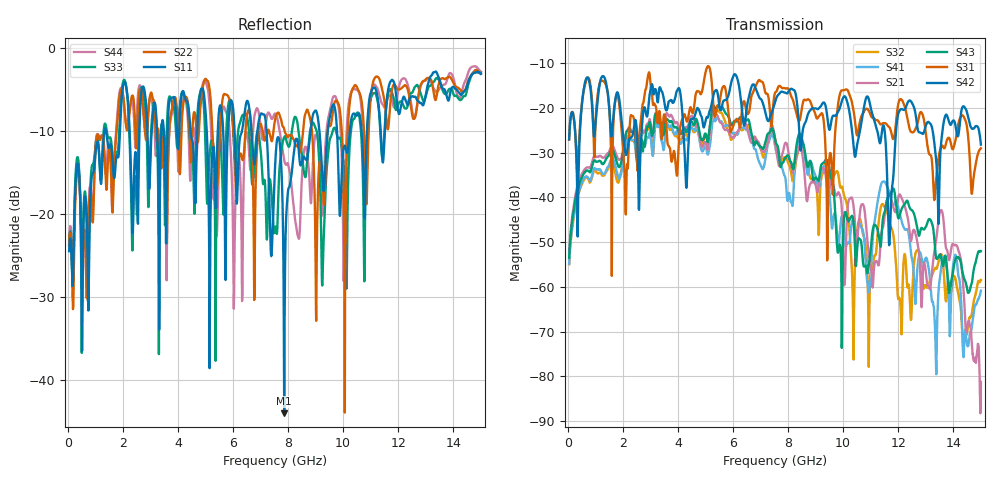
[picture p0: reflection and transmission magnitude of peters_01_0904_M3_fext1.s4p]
# MHZ S RI R 50.00
! FREQ  S11  S12  S13  S14
!  S21  S22  S23  S24
!  S31  S32  S33  S34
!  S41  S42  S43  S44
!  REAL  IMAG  REAL  IMAG  REAL  IMAG  REAL  IMAG
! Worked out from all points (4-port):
!   1496 points, 50 MHz to 15 GHz, reference 50 ohm
!   strongest paths, dB at 50 MHz, 3.79 GHz, 7.53 GHz, 11.27 GHz, 15 GHz:
!     S42: -27.0, -18.6, -18.6, -26.0, -28.2
!     S31: -27.1, -31.7, -16.5, -22.8, -29.0
!     S43: -53.5, -23.1, -27.1, -47.7, -52.0
!     S21: -52.9, -21.9, -28.1, -55.1, -81.3
!     S41: -54.9, -24.4, -28.5, -40.3, -60.9
!     S32: -55.0, -24.9, -26.9, -46.7, -58.5
!   lowest |S11| = -44.0 dB at 7.86 GHz (marker M1), VSWR 1.01, Z = 49.6 + j0.459 ohm
!   |S11| at or under -10 dB: start of sweep to 1.329 GHz; 1.391 GHz to 1.896 GHz (505.2 MHz wide, 30.7 % of centre); 7.216 GHz to 8.812 GHz (1.596 GHz wide, 19.9 % of centre)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
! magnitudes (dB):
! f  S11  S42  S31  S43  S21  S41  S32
! 50 MHz  -24.5  -27.0  -27.1  -53.5  -52.9  -54.9  -55.0
! 3.24 GHz  -9.9  -17.7  -22.1  -21.4  -22.1  -24.0  -23.6
! 7.86 GHz  -44.0  -16.5  -15.5  -31.6  -28.5  -35.0  -31.0
! 10.9 GHz  -8.0  -17.5  -20.3  -56.4  -50.9  -59.9  -61.4
! 11.69 GHz  -4.3  -49.2  -24.4  -39.2  -39.9  -39.3  -45.7
! 13.57 GHz  -4.7  -27.0  -28.6  -53.8  -42.9  -55.3  -52.8
! 15 GHz  -3.1  -28.2  -29.0  -52.0  -81.3  -60.9  -58.5
